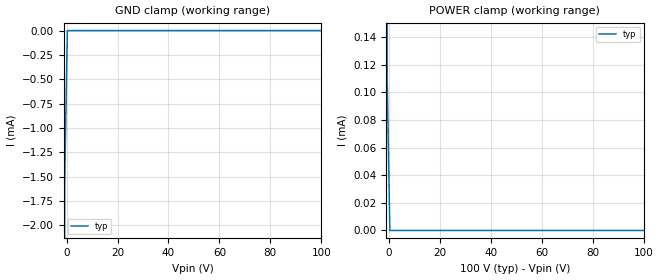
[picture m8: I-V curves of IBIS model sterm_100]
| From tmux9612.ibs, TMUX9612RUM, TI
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| sterm_100
[Model]   sterm_100
Model_type   Terminator
|   typ   min   max
C_comp   1.008417e-11   NA   NA
[Voltage Range]   100   NA   NA
[Temperature Range]   27   NA   NA
[Power Clamp Reference]   100   NA   NA
[GND Clamp Reference]   0   NA   NA
[GND Clamp]
|   Voltage   I(typ)   I(min)   I(max)
-5V       -2.416A    NA         NA
-1.818V   -288.5mA   NA         NA
-757.6mV  -1.579mA   NA         NA
303mV     -1.198nA   NA         NA
100V      2.96nA     NA         NA
[POWER Clamp]
|   Voltage   I(typ)   I(min)   I(max)
-5V       1.055A     NA         NA
-1.818V   191.2mA    NA         NA
-758mV    111.3uA    NA         NA
303mV     2.957nA    NA         NA
100V      -1.21nA    NA         NA
